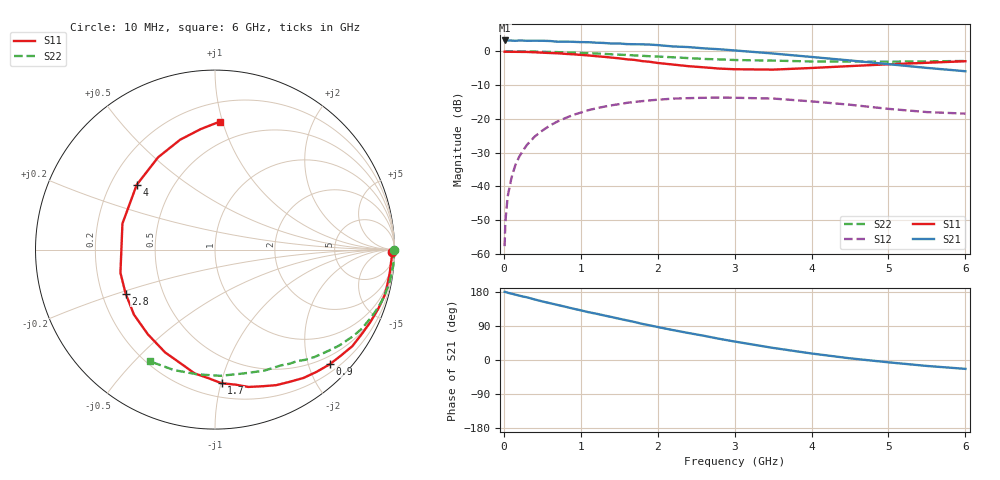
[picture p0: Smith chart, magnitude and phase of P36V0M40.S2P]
! SIEMENS Small Signal Semiconductors
! BFP181
! Si NPN RF Bipolar Junction Transistor in SOT143
! VCE = 6 V  IC = 0.4 mA
! Common Emitter S-Parameters:  March  1996
# GHz  S  MA  R  50
!  f  S11  S21  S12  S22
! GHz  MAG  ANG  MAG  ANG  MAG  ANG  MAG  ANG
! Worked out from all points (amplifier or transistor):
!   36 points, 10 MHz to 6 GHz, reference 50 ohm
!   highest |S21| = 3.2 dB at 10 MHz (marker M1)
!   |S21| within 3 dB of that: start of sweep to 3.023 GHz
!   unconditionally stable (mu >= 1): 3.902 GHz to end of sweep
!   at 250 MHz: K = 0.08, MSG = 16.3 dB, |S12| = -29.4 dB
!   at 1.4 GHz: K = 0.42, MSG = 9.2 dB, |S12| = -16.0 dB
!   at 6 GHz: K = 1.48, MAG = 2.2 dB, |S12| = -18.5 dB
!   S11 on the Smith chart (normalised r, x): 10 MHz: open; 900 MHz: 0.34, -2.37; 1.7 GHz: 0.30, -1.00; 2.8 GHz: 0.30, -0.21; 4 GHz: 0.31, +0.33; 6 GHz: 0.34, +0.98
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0.01  0.9866 -0.7  1.448 179.8  0.0013 84.3  0.9999 -0.2
0.02  0.9869 -1.0  1.438 179.7  0.003 88.7  0.9944 -0.4
0.05  0.9858 -2.4  1.447 177.5  0.0071 92.1  0.9984 -1.3
0.1  0.9825 -5.2  1.441 175.1  0.0135 85.4  0.9978 -2.5
0.15  0.9824 -7.5  1.431 172.5  0.0207 84.4  0.9967 -3.7
0.2  0.9805 -10.1  1.447 169.9  0.0275 82.8  0.9965 -4.9
0.3  0.9786 -15.0  1.43 165.5  0.0411 78.9  0.9937 -7.5
0.5  0.9546 -25.2  1.432 154.6  0.0669 71.5  0.9849 -12.4
0.9  0.9038 -45.0  1.383 135.6  0.1141 57.3  0.9549 -21.8
1.1  0.8686 -55.4  1.365 126.2  0.1343 50.4  0.9367 -26.2
1.5  0.7873 -76.4  1.306 108.9  0.1651 37.7  0.8913 -34.6
1.7  0.7455 -87.2  1.273 100.3  0.1779 32.0  0.8694 -38.4
1.9  0.699 -99.4  1.258 91.3  0.1878 26.2  0.8453 -42.0
2.2  0.6366 -115.9  1.18 78.9  0.1992 18.4  0.8155 -47.2
2.6  0.5791 -141.2  1.106 64.0  0.2048 8.9  0.7709 -53.7
2.8  0.555 -153.8  1.073 55.9  0.2065 4.1  0.7594 -56.9
3  0.5425 -166.2  1.03 48.8  0.2051 -0.5  0.7432 -60.1
3.5  0.5357 164.3  0.928 31.9  0.1997 -10.1  0.728 -68.0
4  0.5662 140.4  0.825 17.2  0.1813 -17.7  0.7075 -77.4
4.5  0.6042 121.6  0.732 4.4  0.1617 -23.3  0.7039 -87.6
5.5  0.676 96.8  0.568 -15.7  0.1259 -22.1  0.7092 -108.9
6  0.7133 87.9  0.507 -23.4  0.1194 -17.3  0.7197 -120.0
